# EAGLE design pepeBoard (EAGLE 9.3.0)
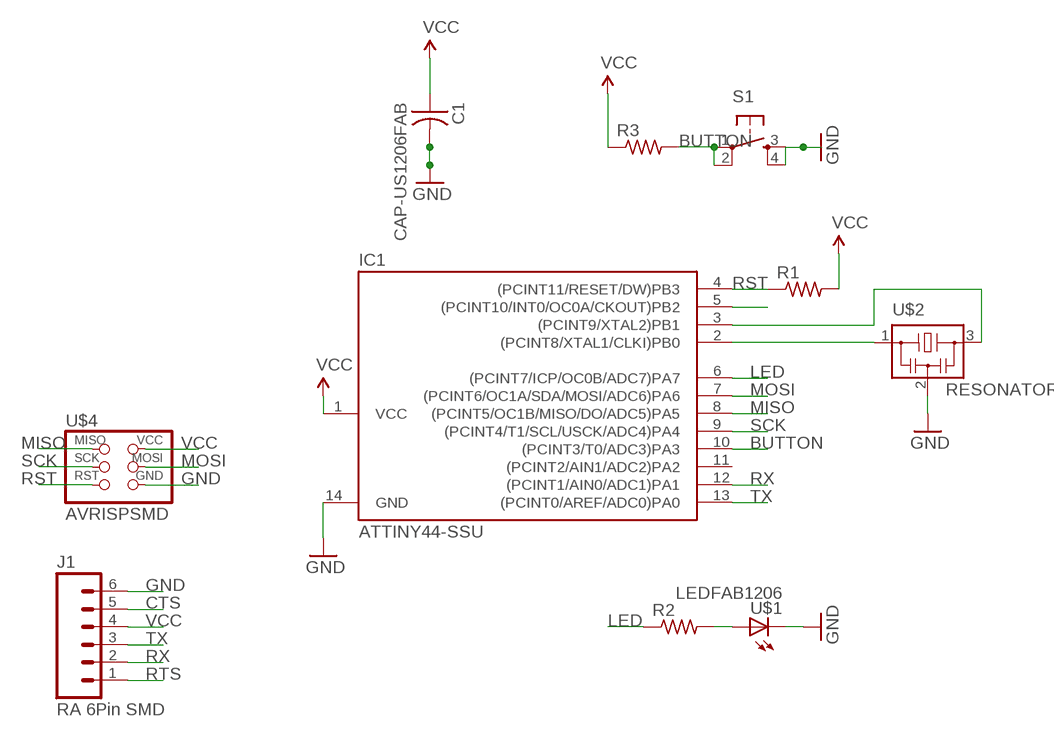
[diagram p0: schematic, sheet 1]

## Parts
C1  CAP-US1206FAB  [C1206FAB]
IC1  ATTINY44-SSU  [SOIC14]
J1  RA 6Pin SMD  M06SMD  [1X06-SMD]
R1  RES-US1206FAB  [R1206FAB]
R2  RES-US1206FAB  [R1206FAB]
R3  RES-US1206FAB  [R1206FAB]
S1  6MM_SWITCH6MM_SWITCH  [6MM_SWITCH]
U$1  LEDFAB1206  [LED1206FAB]
U$2  RESONATOR  [EFOBM]
U$4  AVRISPSMD  [2X03SMD]

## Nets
BUTTON: IC1.10((PCINT3/T0/ADC3)PA3) R3.2 S1.1(P) S1.2(P1)
CTS: J1.5
GND: C1.2 IC1.14(GND) J1.6 S1.3(S) S1.4(S1) U$1.2(C) U$2.2 U$4.6(GND)
LED: IC1.6((PCINT7/ICP/OC0B/ADC7)PA7) R2.1
MISO: IC1.8((PCINT5/OC1B/MISO/DO/ADC5)PA5) U$4.1(MISO)
MOSI: IC1.7((PCINT6/OC1A/SDA/MOSI/ADC6)PA6) U$4.4(MOSI)
N$1: R2.2 U$1.1(A)
N$2: IC1.2((PCINT8/XTAL1/CLKI)PB0) U$2.1
N$6: IC1.3((PCINT9/XTAL2)PB1) U$2.3
N$13: IC1.5((PCINT10/INT0/OC0A/CKOUT)PB2)
RST: IC1.4((PCINT11/RESET/DW)PB3) R1.1 U$4.5(RST)
RTS: J1.1
RX: IC1.12((PCINT1/AIN0/ADC1)PA1) J1.2
SCK: IC1.9((PCINT4/T1/SCL/USCK/ADC4)PA4) U$4.3(SCK)
TX: IC1.13((PCINT0/AREF/ADC0)PA0) J1.3
VCC: C1.1 IC1.1(VCC) J1.4 R1.2 R3.1 U$4.2(VCC)
Unconnected: IC1.11((PCINT2/AIN1/ADC2)PA2)

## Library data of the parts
C1 = fab:CAP-US
IC1 = fab:ATTINY44
J1 = SparkFun-Connectors:M06: Header 6 Standard 6-pin 0.1" header. Use with straight break away headers (SKU : PRT-00116), right angle break away headers (PRT-00553), swiss pins (PRT-00743), machine pins (PRT-00117), and female headers (PRT-00115). Molex polarized connector foot print use with SKU : PRT-08094 with associated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; PROD_ID: CONN-08971
R1 R3 = 01_fab:RES-US: Resistor (US Symbol)
R2 = fab:RES-US: Resistor (US Symbol)
S1 = ng:6MM_SWITCH: OMRON SWITCH
U$1 = 01_fab:LED: LED
U$2 = 01_fab:RESONATOR
U$4 = 01_fab:AVRISP

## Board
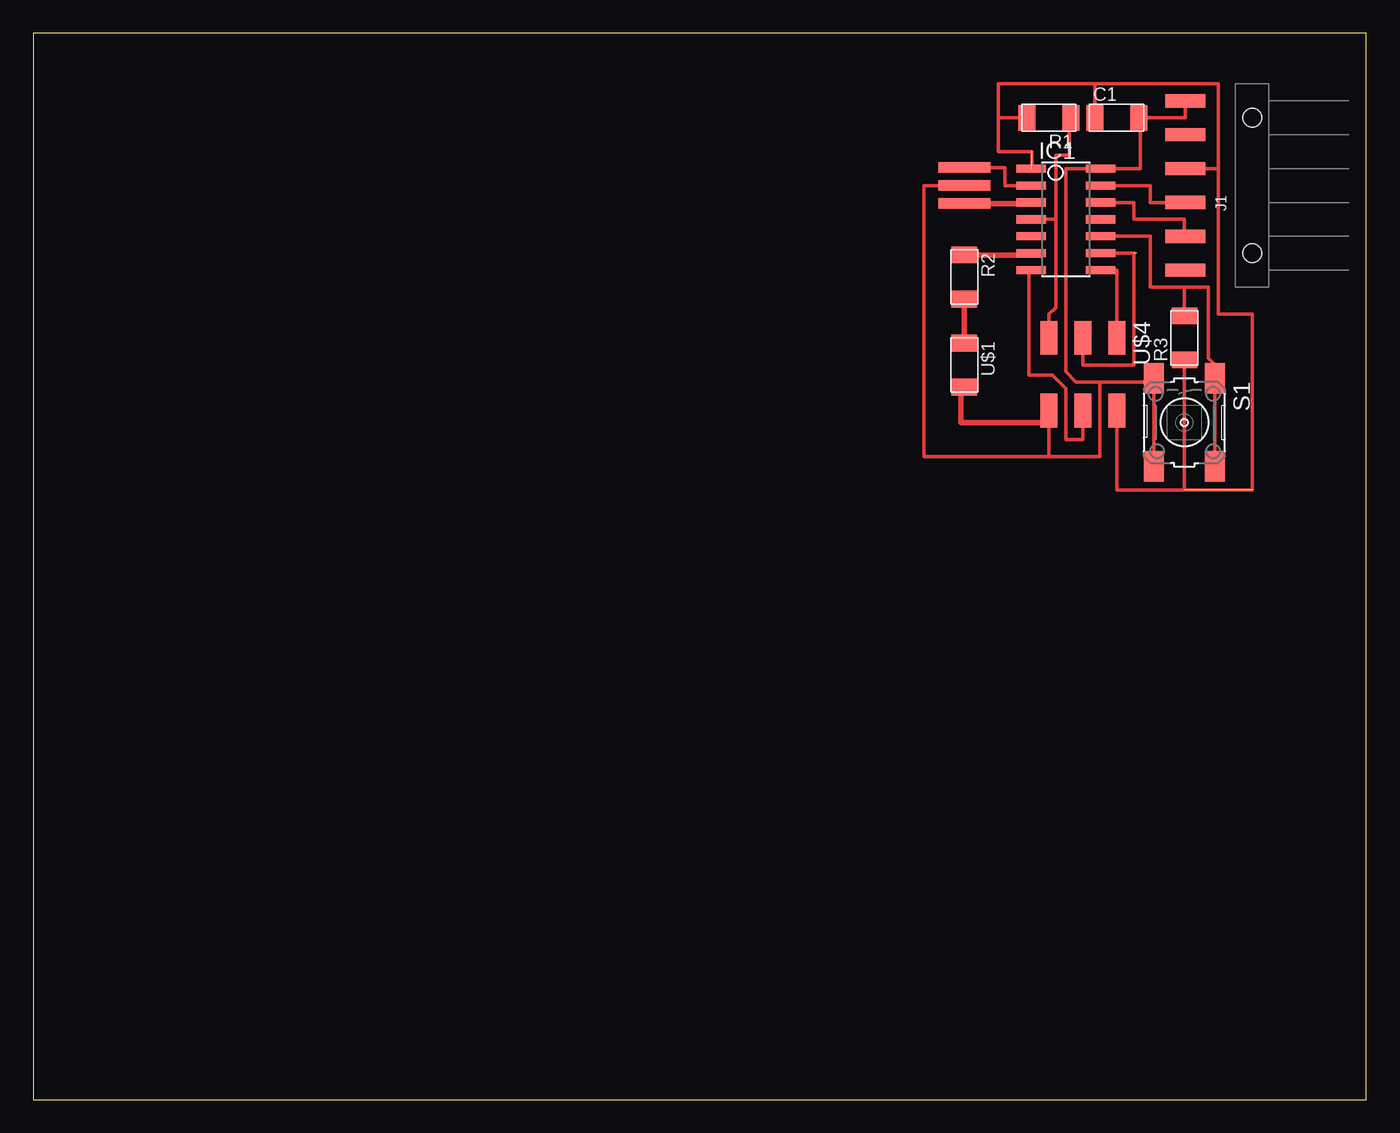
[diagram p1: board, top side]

Size 100 x 80 mm. Coordinates in mm from the lower left corner, seen from the top.
Outline: 0,0 100,0 100,80 0,80 0,0
Copper layers (1*16): Top 0.035mm / dielectric 1.5mm / Bottom 0.035mm
Design rules "pepeBoard": minimum track width 16mil, minimum drill 24mil, track to track 16mil, track to pad 16mil, pad to pad 0.205mm, via to via 0.205mm, smd to smd 16mil, copper to edge 40mil, drill to drill 8mil, minimum pad ring 10mil, minimum via ring 8mil, stop-mask expansion 4mil, vias tented up to drill 0mil, thermal gap 10mil

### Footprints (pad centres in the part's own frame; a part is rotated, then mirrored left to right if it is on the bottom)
C1206FAB = smd 1.27 x 1.905: 1 -1.651,0; 2 1.651,0
SOIC14 = smd 0.61 x 2.21: 1 -3.81,-2.603; 2 -2.54,-2.603; 3 -1.27,-2.603; 4 0,-2.603; 5 1.27,-2.603; 6 2.54,-2.603; 7 3.81,-2.603; 8 3.81,2.603; 9 2.54,2.603; 10 1.27,2.603; 11 0,2.603; 12 -1.27,2.603; 13 -2.54,2.603; 14 -3.81,2.603
1X06-SMD = smd 1 x 3: 1 -6.35,5; 2 -3.81,5; 3 -1.27,5; 4 1.27,5; 5 3.81,5; 6 6.35,5 | hole 1.4: -5.08,0; 5.08,0
R1206FAB = smd 1.27 x 1.905: 1 -1.651,0; 2 1.651,0
6MM_SWITCH = smd 2.286 x 1.524: 1 -3.302,2.286; 2 3.302,2.286; 3 -3.302,-2.286; 4 3.302,-2.286
LED1206FAB = smd 1.27 x 1.905: 1 -1.651,0; 2 1.651,0
EFOBM = smd 0.8 x 3.9: 1 -1.35,0; 2 0,0; 3 1.35,0
2X03SMD = smd 2.54 x 1.27: 1 -2.54,2.54; 2 2.92,2.54; 3 -2.54,0; 4 2.92,0; 5 -2.54,-2.54; 6 2.92,-2.54

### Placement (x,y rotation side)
C1  81.28,73.66 0 top
IC1  77.47,66.04 270 top
J1  91.44,68.58 90 top
R1  76.2,73.66 180 top
R2  69.85,61.72 270 top
R3  86.36,57.15 90 top
S1  86.36,50.8 270 top
U$1  69.85,55.12 270 top
U$2  69.85,68.58 270 top
U$4  78.74,54.61 270 top

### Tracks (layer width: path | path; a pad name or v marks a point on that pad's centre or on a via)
BUTTON
  Top 0.254: 80.01,64.77 IC1.10 83.82,64.77 83.82,60.96 86.36,60.96 | 86.36,60.96 88.14,60.96 88.14,55.63 88.9,54.86 88.9,54.36 S1.1 | 86.36,60.96 R3.2 | S1.1 88.14,54.1 | S1.1 S1.2
GND
  Top 0.254: U$2.2 66.8,68.58 66.8,48.26 76.2,48.26 | 76.2,48.26 76.2,50.8 U$4.6 76.2,52.07 | 76.2,48.26 80.01,48.26 80.01,53.85 | 83.06,73.66 86.44,73.66 J1.6 | C1.2 83.06,73.66 | 83.06,73.66 83.06,69.85 IC1.14 77.47,69.85 77.47,54.61 78.23,53.85 80.01,53.85 | S1.3 84.07,53.85 | 84.07,53.85 80.01,53.85 | S1.4 84.07,53.85
  Top 0.406: U$1.2 69.6,53.47 69.6,50.8 76.2,50.8
LED
  Top 0.254: 75.69,63.37 75.69,63.5 IC1.6
  Top 0.406: R2.1 75.56,63.37 75.69,63.5
MISO
  Top 0.254: IC1.8 81.28,62.23 U$4.1
MOSI
  Top 0.254: 74.93,62.23 IC1.7 74.68,62.23 74.68,54.36 76.45,54.36 77.47,53.34 77.47,49.53 78.74,49.53 U$4.4
N$1
  Top 0.406: U$1.1 R2.2
N$2
  Top 0.254: U$2.1 72.9,69.93 72.9,68.58 IC1.2
N$6
  Top 0.254: 74.87,67.23 IC1.3
  Top 0.406: 74.87,67.23 U$2.3
RST
  Top 0.254: R1.1 77.72,73.61 77.72,70.87 76.71,70.87 76.71,66.04 | 76.35,57.15 U$4.5 | IC1.4 76.71,66.04 | 76.71,57.4 76.2,57.4 U$4.5 | 75.69,57.91 75.69,57.66 U$4.5 | 76.71,66.04 76.71,59.44 76.2,58.93 U$4.5
RX
  Top 0.254: IC1.12 82.55,67.31 82.55,66.04 86.36,66.04 86.36,64.77 J1.2
SCK  (1 unrouted)
  Top 0.254: U$4.3 78.74,55.12 82.55,55.12 82.55,63.5 IC1.9
TX
  Top 0.254: IC1.13 83.82,68.58 83.82,67.31 J1.3
VCC  (3 unrouted)
  Top 0.254: J1.4 88.9,69.85 | 86.36,45.72 91.44,45.72 91.44,58.93 88.9,58.93 88.9,69.85 | 86.36,45.72 81.28,45.72 U$4.2 | 79.63,76.2 72.39,76.2 72.39,73.66 | 79.63,76.2 C1.1 | IC1.1 74.93,69.85 74.93,71.12 72.39,71.12 72.39,73.66 | 72.39,73.66 R1.2 | 79.63,76.2 88.9,76.2 88.9,69.85 | R3.1 86.36,45.72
